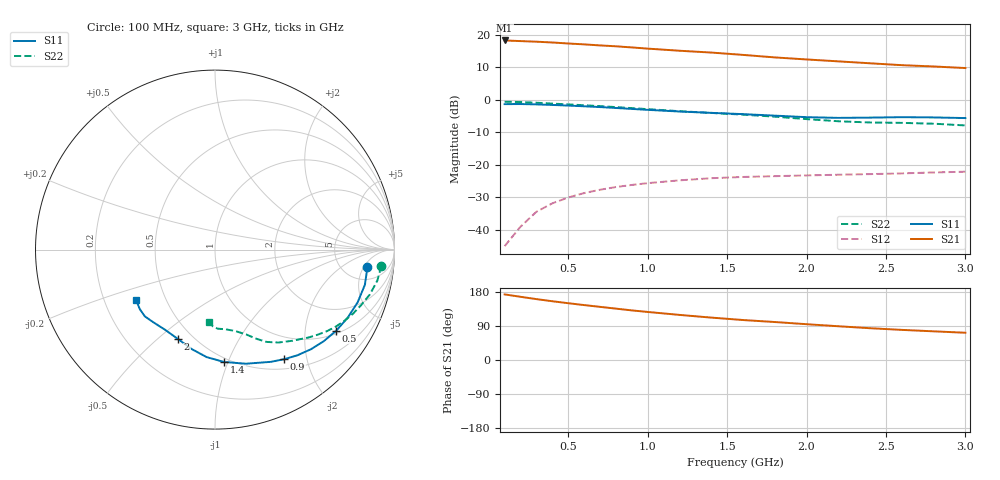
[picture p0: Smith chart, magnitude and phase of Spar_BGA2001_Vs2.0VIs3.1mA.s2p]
! Filename: 2G1.001
! Title: BGA2001 X0297-20 HFE=80
! Bias: Vce=2.0V,Ic=3.1mA
! Company: NXP Semiconductors NL
! User: Quality&Reliability T&D
! Measure time: 23 Oct 1998 / 09:19:30
#  MHz  S  MA  R 50
! Freq  S11  S21  S12  S22  :
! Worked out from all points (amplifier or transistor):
!   20 points, 100 MHz to 3 GHz, reference 50 ohm
!   highest |S21| = 18.2 dB at 100 MHz (marker M1)
!   |S21| within 3 dB of that: start of sweep to 1.153 GHz
!   unconditionally stable (mu >= 1): 2.373 GHz to end of sweep
!   at 400 MHz: K = 0.19, MSG = 24.7 dB, |S12| = -31.8 dB
!   at 1.2 GHz: K = 0.46, MSG = 19.9 dB, |S12| = -24.7 dB
!   at 3 GHz: K = 1.18, MAG = 13.4 dB, |S12| = -22.1 dB
!   S11 on the Smith chart (normalised r, x): 100 MHz: 8, -6; 500 MHz: 1.10, -2.92; 900 MHz: 0.64, -1.63; 1.4 GHz: 0.47, -0.97; 2 GHz: 0.42, -0.59; 3 GHz: 0.34, -0.26
100  0.855 -6.4  8.11 173.1  0.005657 59.3  0.9313 -5.6
200  0.8579 -13.2  7.93 166.8  0.01125 81.7  0.9206 -10.9
300  0.8472 -20.4  7.764 160.7  0.01905 79.4  0.8984 -16.1
400  0.8308 -27.2  7.546 155.1  0.02567 74.9  0.8714 -20.8
500  0.8126 -33.7  7.286 149.9  0.03155 70.9  0.847 -25.0
600  0.7924 -40.0  7.063 145.0  0.03687 67.3  0.8218 -29.0
700  0.771 -46.0  6.81 140.3  0.04152 64.1  0.7967 -32.8
800  0.7468 -52.0  6.598 135.6  0.04569 61.1  0.77 -36.3
900  0.7219 -57.8  6.341 130.9  0.0492 58.4  0.7427 -39.7
1000  0.6988 -63.5  6.079 126.8  0.0524 56.0  0.7163 -43.1
1200  0.6589 -74.8  5.642 119.0  0.05789 51.9  0.6666 -49.6
1400  0.6281 -85.4  5.29 111.9  0.06243 48.5  0.6267 -55.7
1600  0.6006 -94.5  4.87 105.5  0.06524 46.5  0.5897 -60.7
1800  0.5696 -103.0  4.457 100.2  0.0671 45.7  0.5491 -65.0
2000  0.5396 -112.3  4.144 94.5  0.0689 44.3  0.5039 -69.8
2200  0.5262 -122.1  3.876 89.1  0.07058 43.0  0.4668 -76.1
2400  0.5312 -130.4  3.62 83.9  0.07217 42.7  0.447 -82.9
2600  0.5394 -136.4  3.387 79.5  0.07399 44.0  0.4409 -88.1
2800  0.5346 -141.5  3.235 75.7  0.07649 44.2  0.4284 -91.5
3000  0.5224 -147.3  3.06 71.9  0.07856 45.0  0.4027 -95.1
